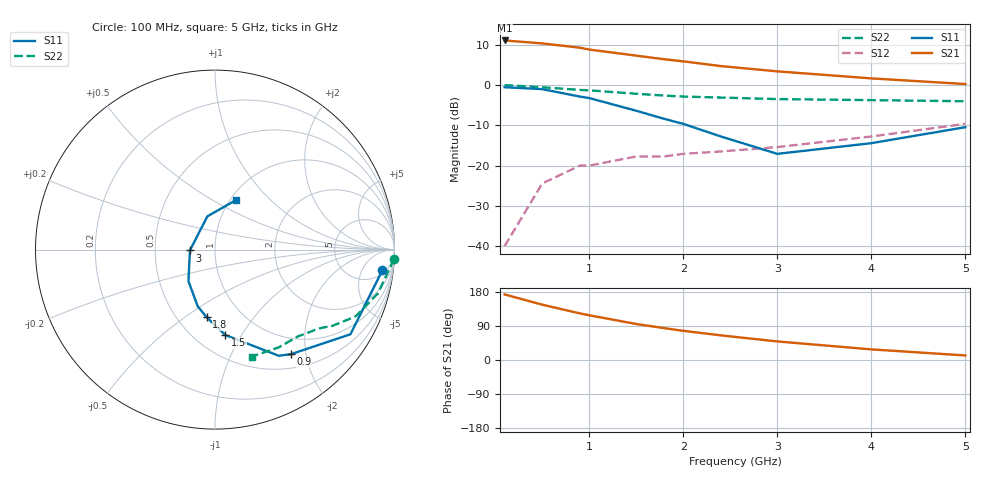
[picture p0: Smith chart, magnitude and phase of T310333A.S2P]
!AT-31033
!S and NOISE PARAMETERS at Vce=2.7V  Ic=1mA.  LAST UPDATED 06-23-94
# ghz s ma r 50
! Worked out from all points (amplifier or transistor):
!   11 points, 100 MHz to 5 GHz, reference 50 ohm
!   highest |S21| = 11.1 dB at 100 MHz (marker M1)
!   |S21| within 3 dB of that: start of sweep to 1.245 GHz
!   unconditionally stable (mu >= 1): 2.286 GHz to 4.204 GHz
!   at 500 MHz: K = 0.26, MSG = 17.4 dB, |S12| = -24.4 dB
!   at 1.8 GHz: K = 0.88, MSG = 12.1 dB, |S12| = -17.7 dB
!   at 5 GHz: K = 0.89, MSG = 4.9 dB, |S12| = -9.6 dB
!   lowest NFmin = 0.50 dB at 500 MHz
!   S11 on the Smith chart (normalised r, x): 100 MHz: 7, -13; 900 MHz: 0.72, -1.73; 1.5 GHz: 0.69, -0.86; 1.8 GHz: 0.69, -0.61; 3 GHz: 0.75, -0.01; 5 GHz: 1.06, +0.65
0.1  0.94 -7.0  3.58 173.0  0.01 86.0  0.999 -3.0
0.5  0.89 -32.0  3.29 146.0  0.06 70.0  0.94 -15.0
0.9  0.72 -54.0  2.91 123.0  0.1 58.0  0.87 -25.0
1  0.69 -59.0  2.76 118.0  0.1 56.0  0.86 -26.0
1.5  0.48 -83.0  2.32 95.0  0.13 48.0  0.78 -33.0
1.8  0.38 -97.0  2.09 84.0  0.13 46.0  0.74 -36.0
2  0.33 -107.0  1.97 77.0  0.14 45.0  0.72 -38.0
2.4  0.23 -130.0  1.72 65.0  0.15 46.0  0.7 -41.0
3  0.14 -178.0  1.48 49.0  0.17 48.0  0.67 -46.0
4  0.19 103.0  1.21 28.0  0.23 51.0  0.65 -57.0
5  0.3 67.0  1.03 12.0  0.33 47.0  0.63 -71.0
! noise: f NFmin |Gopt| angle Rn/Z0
0.5  0.5  0.9  12  0.7
0.9  0.6  0.82  28  0.6
1.8  1.1  0.57  68  0.38
2.4  1.6  0.41  100  0.22
